FUNCTION F_ReplaceByString : T_MaxString			(* Find first content & replace *)
VAR_INPUT
		sSource			: T_MaxString;	(* Data Source *)
		sFindContent	: T_MaxString;	(* Find feature *)
		sReplaceContent	: T_MaxString;	(* replace content *)
END_VAR
VAR
	i : INT;	

END_VAR

(*
F_ReplaceByString := sSource; 
*)
IF find(sSource , sFindContent)> 0  THEN
	F_ReplaceByString := sSource; 
i := 	find(sSource , sFindContent);
	F_ReplaceByString := REPLACE(sSource , sReplaceContent ,Len(sFindContent) , find(sSource,sFindContent));
END_IF

END_FUNCTION
